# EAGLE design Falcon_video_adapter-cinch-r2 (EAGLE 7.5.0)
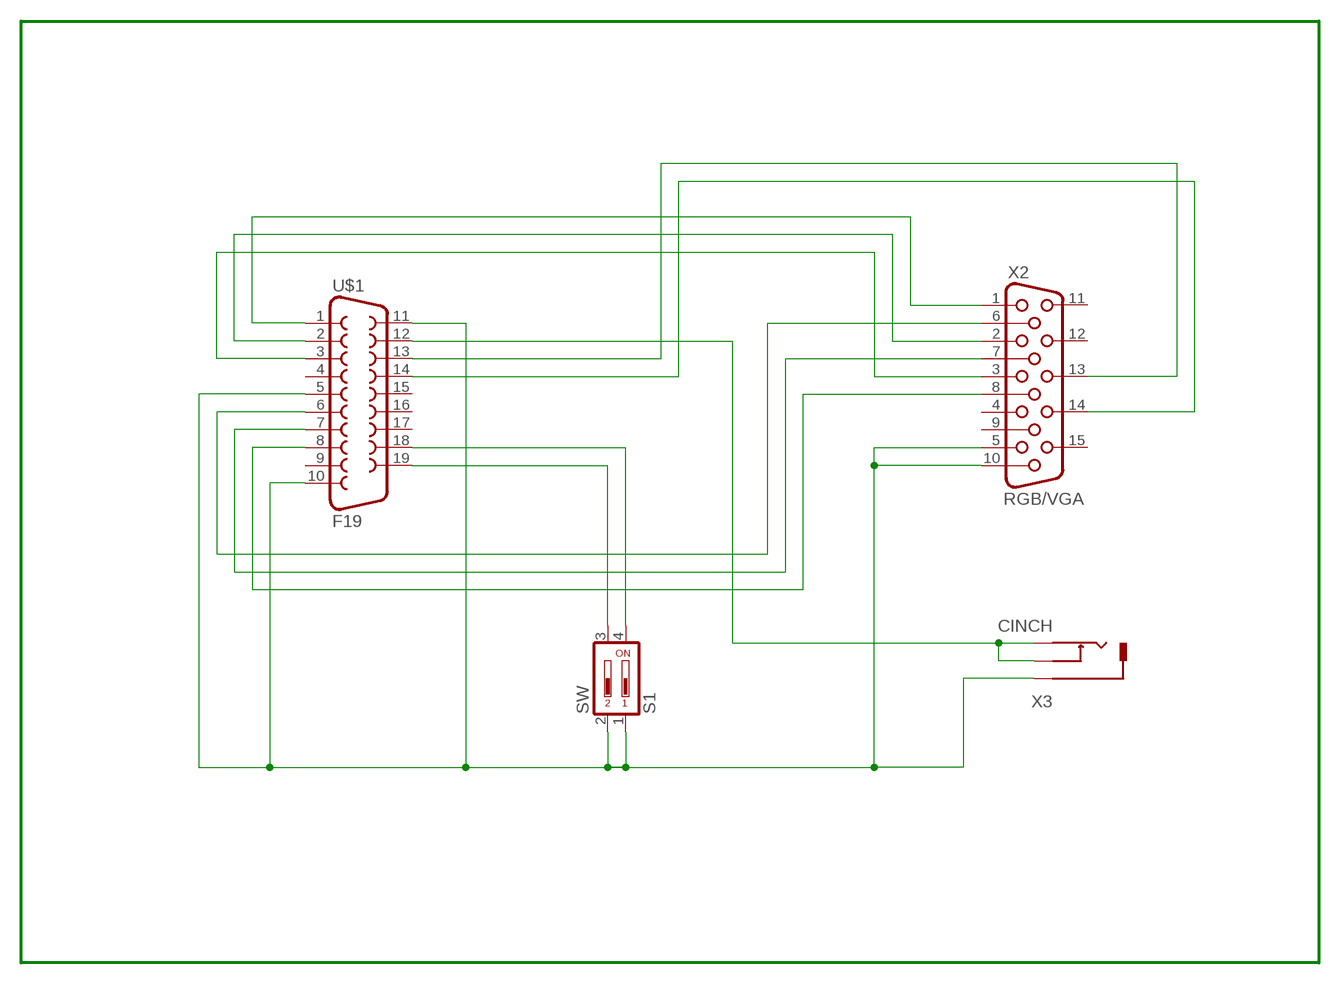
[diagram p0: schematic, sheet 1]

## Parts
S1  SW  DIP02YL  [DIP02YL]
U$1  F19  [F19D]
X2  RGB/VGA  HF15H  [HDF15H]
X3  CINCH  [SJC-0358]

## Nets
B: U$1.3 X2.3
COMPOSITE: U$1.12 X3.1 X3.3
G: U$1.2 X2.2
GND: S1.1 S1.2 U$1.5 U$1.10 U$1.11 X2.5 X2.10 X3.2
GND_B: U$1.8 X2.8
GND_G: U$1.7 X2.7
GND_R: U$1.6 X2.6
HS: U$1.14 X2.14
M0: S1.3 U$1.19
M1: S1.4 U$1.18
R: U$1.1 X2.1
VS: U$1.13 X2.13
Unconnected: U$1.4 U$1.9 U$1.15 U$1.16 U$1.17 X2.4 X2.9 X2.11 X2.12 X2.15

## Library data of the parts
S1 = switch-dil:DIP02YL: DIL/CODE SWITCH; OC_FARNELL: unknown; OC_NEWARK: unknown
U$1 = con-subd:F19
X2 = con-subd:HF15: SUB-D; OC_FARNELL: unknown; OC_NEWARK: unknown
X3 = cinch:CINCH: Cinch Connector ( RCA Jack )

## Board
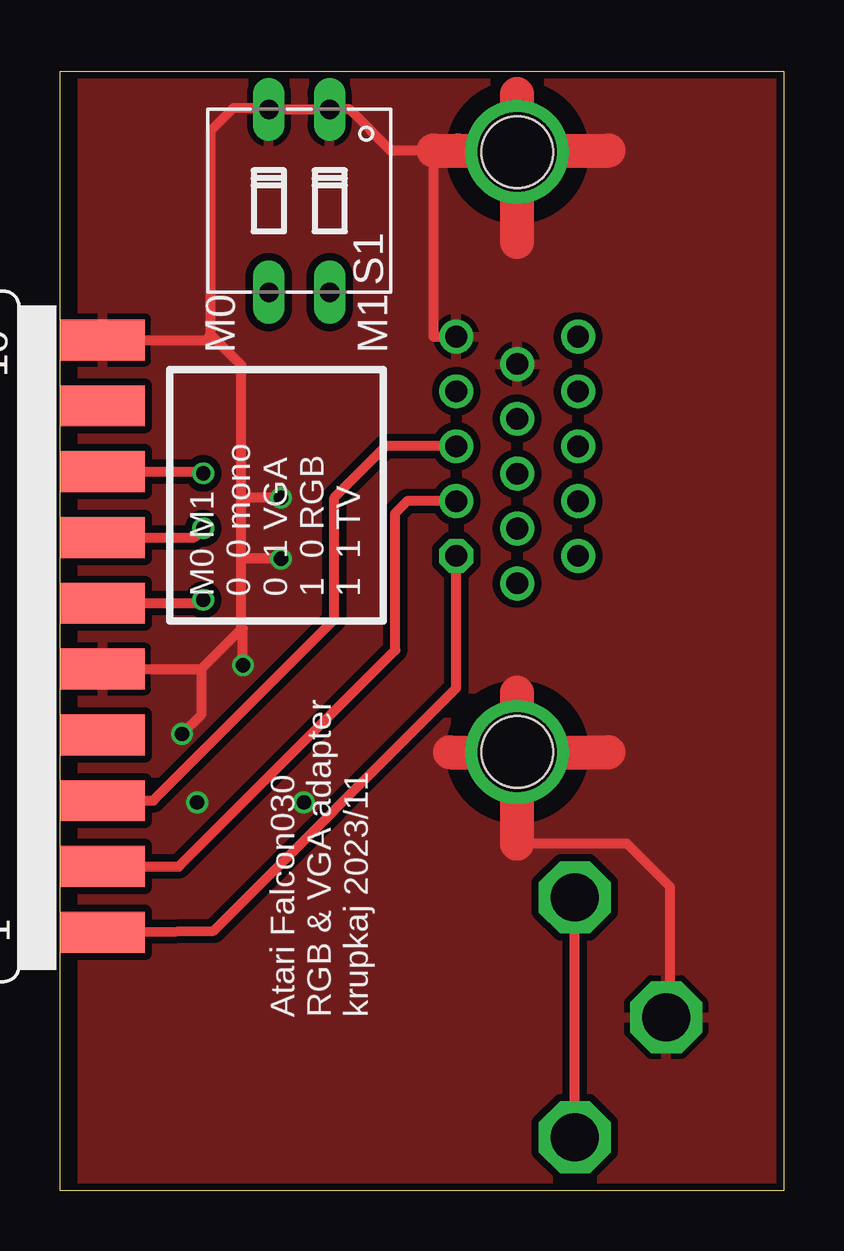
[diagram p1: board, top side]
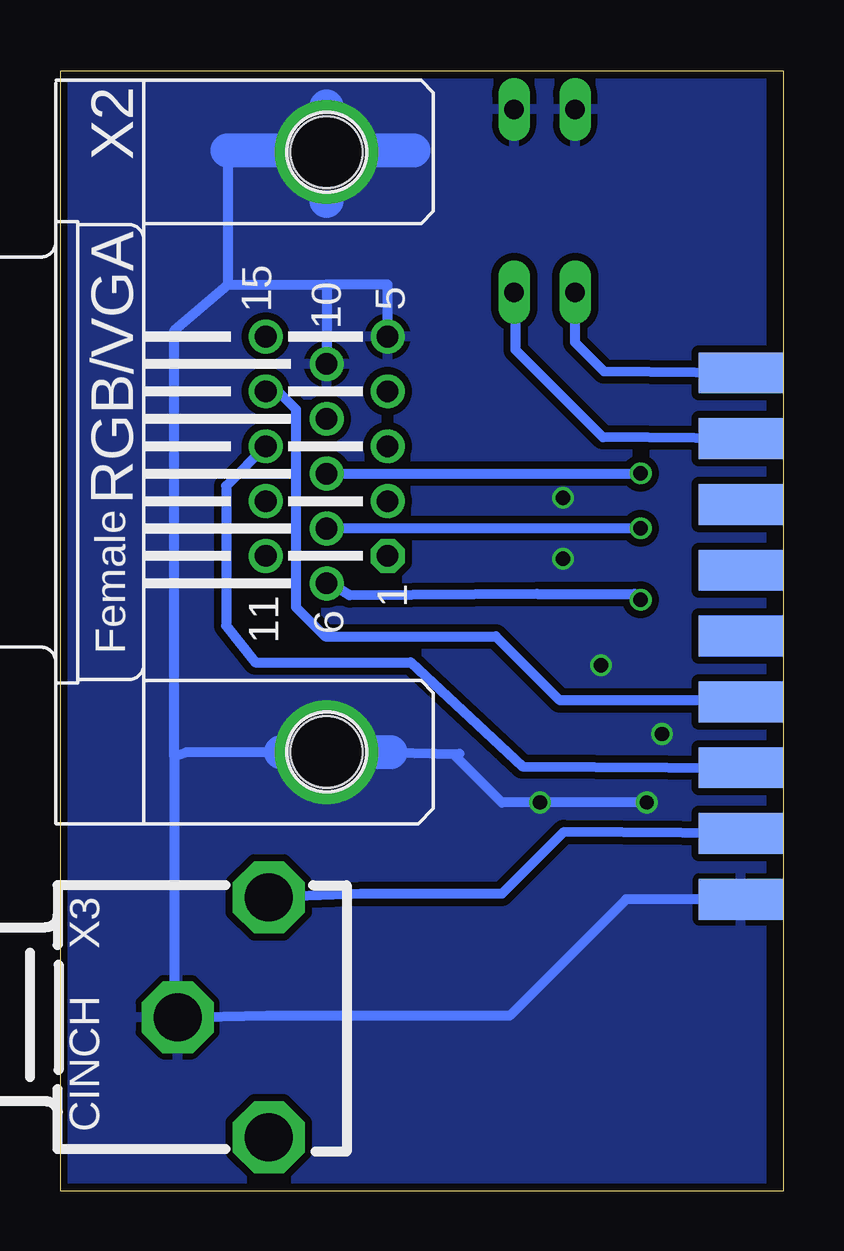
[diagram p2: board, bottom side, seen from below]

Size 30.16 x 46.67 mm. Coordinates in mm from the lower left corner, seen from the top.
Outline: 0,46.67 30.16,46.67 30.16,0 0,0 0,46.67
Copper layers (1*16): Top 0.035mm / dielectric 1.5mm / Bottom 0.035mm
Design rules "SeeedStudio_2layer_DRU_no_angle_20140221": minimum track width 6mil, minimum drill 12mil, track to track 6mil, track to pad 6mil, pad to pad 6mil, via to via 6mil, smd to smd 0mil, copper to edge 10mil, drill to drill 10mil, minimum pad ring 10mil, minimum via ring 6mil, stop-mask expansion 2mil, vias tented up to drill 100mil, thermal gap 10mil

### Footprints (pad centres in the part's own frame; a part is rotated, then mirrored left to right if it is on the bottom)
DIP02YL = drill 0.813 long: 1 -1.27,-3.81; 2 1.27,-3.81; 3 1.27,3.81; 4 -1.27,3.81
F19D = smd 1.7 x 3.5: 1 -16.459,-6.045; 2 -13.716,-6.045; 3 -10.973,-6.045; 4 -8.23,-6.045; 5 -5.486,-6.045; 6 -2.743,-6.045; 7 0,-6.045; 8 2.743,-6.045; 9 5.486,-6.045; 10 8.23,-6.045 | smd 1.7 x 3.5 bottom: 11 -15.088,-6.045; 12 -12.344,-6.045; 13 -9.601,-6.045; 14 -6.858,-6.045; 15 -4.115,-6.045; 16 -1.372,-6.045; 17 1.372,-6.045; 18 4.115,-6.045; 19 6.858,-6.045
HDF15H = drill 0.9 octagon: 1 4.329,2.54 | drill 0.9: 2 2.043,2.54; 3 -0.243,2.54; 4 -2.529,2.54; 5 -4.815,2.54; 6 5.472,0; 7 3.186,0; 8 0.9,0; 9 -1.386,0; 10 -3.672,0; 11 4.329,-2.54; 12 2.043,-2.54; 13 -0.243,-2.54; 14 -2.529,-2.54; 15 -4.815,-2.54 | hole 3: -12.5,0; 12.5,0
SJC-0358 = drill 2 octagon: 1 8.96,5; 2 5.16,0; 3 8.96,-5

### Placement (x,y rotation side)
S1  9.97,41.27 180 top
U$1  -4.25,27.24 90 top
X2  19.05,30.8 270 bottom
X3  30.42,7.24 0 bottom

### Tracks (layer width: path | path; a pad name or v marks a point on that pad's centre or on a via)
B
  Top 0.406: U$1.3 3.89,16.27 11.43,23.81 11.43,28.89 13.58,31.04 X2.3
COMPOSITE
  Top 0.406: X3.3 X3.1
  Bottom 0.406: U$1.12 9.17,14.96 11.75,12.38 17.63,12.38 X3.1
G
  Top 0.406: U$1.2 4.95,13.53 13.97,22.54 13.97,28.26 14.47,28.75 X2.2
GND  (via drill 0.6, 3.3 pad 3.81)
  Top 0.406: v19.05,43.31 16.57,43.37 16.64,43.37 | 16.51,43.56 15.56,43.37 | 6.29,35.69 6.29,44.2 7.24,45.15 8.64,45.15 S1.2 S1.1 12.06,45.09 13.78,43.37 15.56,43.37 | U$1.5 5.88,21.76 | 5.88,21.76 7.56,23.43 7.56,23.49 | 7.56,23.49 7.56,26.35 | 7.56,26.35 7.56,28.57 | 7.56,28.57 7.56,34.42 6.29,35.69 | U$1.10 6.07,35.47 6.29,35.69 | 5.88,21.76 5.88,19.85 v5.08,19.05 | 19.05,14.48 23.62,14.48 25.4,12.7 25.4,7.38 X3.2 | 15.56,43.37 15.56,35.61 X2.5 | v9.21,28.89 7.87,28.89 7.56,28.57 | v9.21,26.35 7.56,26.35 | v7.62,21.91 7.62,23.43 7.56,23.49
  Top 1.422: 15.56,43.37 16.57,43.37 22.86,43.37 | 19.05,39.56 v19.05,43.31 19.05,45.72 | 19.05,14.48 19.05,20.76 | 16.26,18.29 22.86,18.29
  Bottom 0.406: U$1.11 6.58,12.15 11.43,7.3 21.51,7.3 21.53,7.32 X3.2 25.4,7.38 25.4,18.1 | v5.71,16.19 v10.16,16.19 11.75,16.19 13.65,18.1 13.53,18.22 16.38,18.29 | 23.18,43.37 23.18,37.78 | 23.18,37.78 19.05,37.78 | 19.05,37.78 X2.10 | 25.4,18.1 25.4,35.88 23.18,37.78 | 20.95,18.29 24.89,18.29 25.4,18.1 | X2.5 16.51,37.78 19.05,37.78
  Bottom 1.422: 16.38,18.29 20.95,18.29 | 19.05,41.28 19.05,45.21 | 15.43,43.37 23.18,43.37
  other vias: 19.05,18.29
  pour Top (isolate 0.305): 34.93,-1.9 0.95,-1.9 0.95,49.85 34.93,49.85
  pour Bottom (isolate 0.305): 32.07,47.62 0.95,47.62 0.95,-4.76 32.07,-4.76
GND_B  (via drill 0.6)
  Top 0.406: U$1.8 5.89,29.98 v5.97,29.91
  Bottom 0.406: X2.8 19.04,29.91 v5.97,29.91
GND_G  (via drill 0.6)
  Top 0.406: U$1.7 5.59,27.24 v5.97,27.62
  Bottom 0.406: X2.7 v5.97,27.62
GND_R  (via drill 0.6)
  Top 0.406: U$1.6 5.83,24.5 v5.97,24.64
  Bottom 0.406: X2.6 18.91,25.33 18.1,24.83 10.29,24.89 6.22,24.89 v5.97,24.64
HS
  Bottom 0.406: U$1.14 0.58,20.45 9.33,20.45 12,23.11 19.11,23.11 20.32,24.32 20.32,32.58 21.07,33.33 X2.14
M0
  Bottom 0.406: U$1.19 7.49,34.16 8.7,35.37 S1.3
M1
  Bottom 0.406: U$1.18 7.54,31.42 11.18,35.05 11.18,37.4 S1.4
R
  Top 0.406: U$1.1 6.4,10.85 16.51,20.96 X2.1
VS
  Bottom 0.406: X2.13 23.24,29.39 23.24,23.56 22.04,22.03 15.56,22.03 10.91,17.7 U$1.13

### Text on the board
tNames: M0 | M1 | M0 M1 / 0 0 mono / 0 1 VGA / 1 0 RGB / 1 1 TV | Atari Falcon030 / RGB & VGA adapter / krupkaj 2023/11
